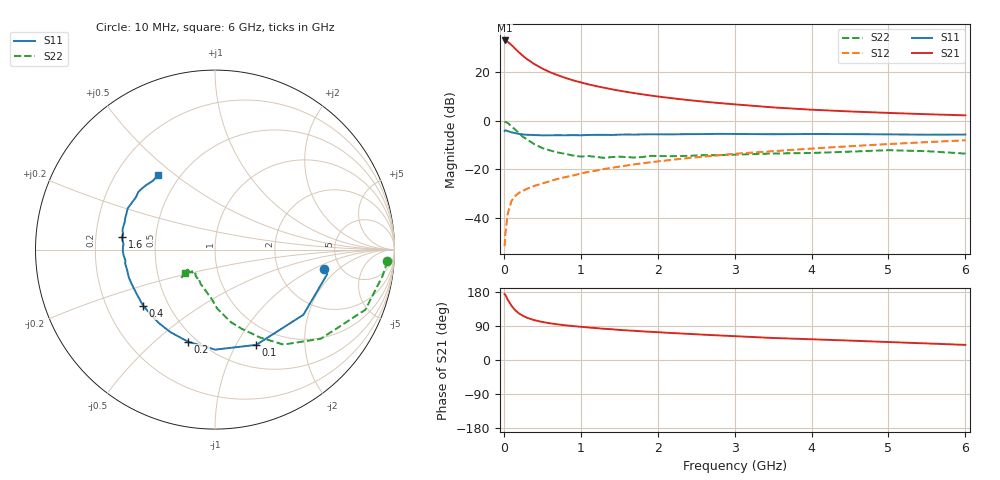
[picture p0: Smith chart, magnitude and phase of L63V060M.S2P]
!  INFINEON TECHNOLOGIES Small Signal Semiconductors
! BFR380L3 , Si-NPN RF-Transistor in TSLP-3-1
!  Vce=3 V,  Ic=60 mA
! Common Emitter S-Parameters:  07. March 2005
#  GHz  S  MA  R  50
! f  S11  S21  S12  S22
! GHz  Mag  Ang  Mag  Ang  Mag  Ang  Mag  Ang
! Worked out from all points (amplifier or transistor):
!   36 points, 10 MHz to 6 GHz, reference 50 ohm
!   highest |S21| = 33.1 dB at 10 MHz (marker M1)
!   |S21| within 3 dB of that: start of sweep to 135.1 MHz
!   unconditionally stable (mu >= 1): 1.372 GHz to 4.835 GHz
!   at 250 MHz: K = 0.51, MSG = 27.8 dB, |S12| = -28.9 dB
!   at 1.4 GHz: K = 1.00, MAG = 15.9 dB, |S12| = -19.4 dB
!   at 6 GHz: K = 0.98, MSG = 5.2 dB, |S12| = -8.1 dB
!   S11 on the Smith chart (normalised r, x): 10 MHz: 3.75, -1.32; 100 MHz: 0.76, -1.21; 200 MHz: 0.45, -0.65; 400 MHz: 0.36, -0.31; 1.6 GHz: 0.31, +0.06; 6 GHz: 0.38, +0.43
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0.01  0.6191 -10.1  45.33 174.0  0.0026 78.6  0.9631 -3.9
0.02  0.6397 -12.4  44.98 171.8  0.0046 85.7  0.9457 -8.8
0.05  0.6118 -36.4  42.55 159.4  0.0122 74.8  0.902 -21.8
0.1  0.5784 -66.6  36.43 143.0  0.0223 64.9  0.7711 -40.1
0.15  0.5573 -89.9  30.42 130.8  0.0284 58.2  0.6523 -54.2
0.2  0.5348 -106.2  25.45 122.4  0.033 55.5  0.55 -62.9
0.25  0.5228 -118.5  21.73 116.4  0.036 54.1  0.4647 -71.4
0.3  0.5149 -127.9  18.72 111.6  0.0396 54.3  0.4142 -77.6
0.4  0.5084 -141.8  14.66 104.9  0.0457 54.7  0.3267 -88.1
0.5  0.5014 -150.9  11.98 100.4  0.051 57.6  0.2746 -94.0
0.6  0.5024 -157.7  10.05 96.8  0.0568 59.3  0.2451 -100.3
0.7  0.5046 -162.1  8.712 94.1  0.0635 60.9  0.2221 -106.5
0.9  0.5066 -171.2  6.828 89.5  0.0744 63.3  0.1924 -116.7
1.1  0.5102 -176.4  5.648 85.8  0.0885 65.1  0.1875 -121.9
1.3  0.5131 178.3  4.819 82.4  0.1012 65.8  0.1721 -129.4
1.6  0.5228 172.1  3.933 78.1  0.1197 66.5  0.1783 -136.5
2.2  0.5259 163.1  2.901 71.0  0.1577 67.0  0.1865 -138.0
2.8  0.5376 154.8  2.321 64.8  0.1951 66.6  0.1952 -143.7
3.5  0.5285 146.4  1.888 58.1  0.2363 64.4  0.2117 -141.8
4.5  0.5312 140.5  1.558 51.2  0.2992 62.4  0.2311 -140.8
5.5  0.5166 132.3  1.366 43.7  0.3632 58.5  0.2364 -140.3
6  0.5205 127.5  1.295 39.9  0.3956 56.2  0.2107 -142.5
